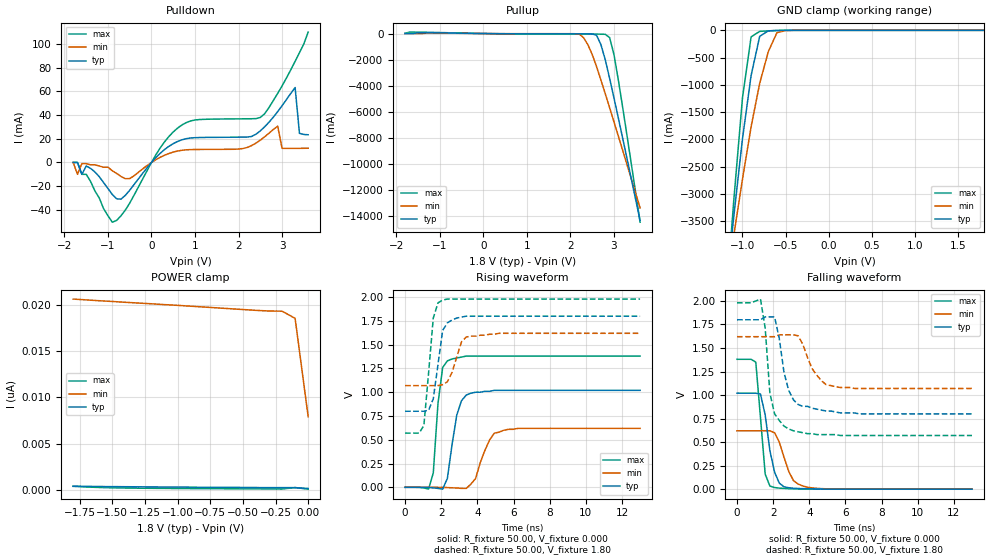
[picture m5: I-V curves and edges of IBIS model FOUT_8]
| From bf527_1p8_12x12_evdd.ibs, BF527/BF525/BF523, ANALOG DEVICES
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|   Model prw0408swcdg_3v_25
[Model]   FOUT_8
Model_type   I/O
Polarity   Non-Inverting
Enable   Active-Low
Vinl =   0.70V
Vinh =   1.00V
Vmeas =   1.20V
Cref =  50.00pF
Rref =   1.00M
Vref =  0.000V
C_comp   4.55pF   4.10pF   5.01pF
[Temperature Range]   25.00   0.12k   -40.00
[Voltage Range]   1.80V   1.62V   1.98V
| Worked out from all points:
|   slope of the pulldown table from 0 to 0.27 V, typ, clamps not added: 27.1 ohm
|   slope of the pullup table from 0 to 0.27 V, typ, clamps not added: 26.9 ohm
|   GND clamp passes 1 mA (typ) near -0.53 V on its own axis
|   rising waveform, R_fixture 50.00, V_fixture 0.000: 20-80 % time 537ps typ, 722ps min, 368ps max; typ from 0 V to 1.02 V
|   rising waveform, R_fixture 50.00, V_fixture 1.80: 20-80 % time 433ps typ, 566ps min, 388ps max; typ from 0.8 V to 1.8 V
|   falling waveform, R_fixture 50.00, V_fixture 0.000: 20-80 % time 524ps typ, 689ps min, 361ps max; typ from 1.02 V to 0 V
|   falling waveform, R_fixture 50.00, V_fixture 1.80: 20-80 % time 650ps typ, 854ps min, 454ps max; typ from 1.8 V to 0.8 V
[Pulldown]
| voltage   I(typ)   I(min)   I(max)
-1.8V     0A         0A         0A
-1.7V     0A         -10mA      0A
-1.6V     -10mA      -1mA       -10mA
-1.4V     -5mA       -2mA       -16mA
-800mV    -30.7mA    -9.3mA     -48.85mA
500mV     15.88mA    8.74mA     25.76mA
2.5V      26.66mA    18.81mA    37.95mA
2.9V      42.92mA    30.63mA    58.28mA
3V        47.86mA    11.94mA    64.57mA
3.3V      63.22mA    11.88mA    85.31mA
3.4V      24.55mA    11.91mA    92.64mA
3.6V      23.36mA    12mA       110mA
[Pullup]
| voltage   I(typ)   I(min)   I(max)
-1.8V     1.53mA     550uA      10.64mA
-1.6V     3.01mA     560uA      110mA
2.2V      -22.71mA   -39.8mA    -37.75mA
2.3V      -23.18mA   -310mA     -37.82mA
2.4V      -25.42mA   -850mA     -37.94mA
2.6V      -130mA     -2.54A     -42.67mA
2.7V      -850mA     -3.56A     -49.74mA
2.8V      -2.01A     -4.61A     -61.07mA
2.9V      -3.43A     -5.68A     -310mA
3V        -4.93A     -6.76A     -1.61A
3.1V      -6.46A     -7.85A     -3.55A
3.6V      -14.31A    -13.35A    -14.44A
[GND_clamp]
| voltage   I(typ)   I(min)   I(max)
-1.8V     -14.28A    -11.35A    -18.41A
-1.2V     -4.9A      -4.81A     -5.19A
-1.1V     -3.4A      -3.75A     -3.1A
-1V       -1.99A     -2.73A     -1.24A
-900mV    -830mA     -1.77A     -120mA
-800mV    -110mA     -970mA     -19.21mA
-700mV    -9.89mA    -390mA     -9.78mA
-600mV    -2.57mA    -42.87mA   -3.5mA
-500mV    -460uA     -4.38mA    -550uA
1.8V      170pA      19.28nA    82.46pA
[POWER_clamp]
| voltage   I(typ)   I(min)   I(max)
-1.8V     420pA      20.63nA    400pA
-1.5V     370pA      20.37nA    240pA
-1.3V     350pA      20.2nA     200pA
-400mV    270pA      19.41nA    130pA
-200mV    260pA      19.32nA    110pA
-100mV    260pA      18.55nA    270pA
0V        170pA      7.92nA     95.65pA
[Ramp]
| variable   typ   min   max
dV/dt_r   0.61/0.49n   0.37/0.70n   0.83/0.31n
dV/dt_f   0.60/0.62n   0.33/0.81n   0.84/0.40n
R_load = 50.00
[Rising Waveform]
R_fixture = 50.00
V_fixture = 0.000
V_fixture_min = 0.000
V_fixture_max = 0.000
L_fixture = 0.000H
C_fixture = 0.000F
| time   V(typ)   V(min)   V(max)
0s        0V         0V         0V
1.3ns     -1.27mV    63.15uV    -18.06mV
1.56ns    -6.38mV    20.98uV    150mV
1.82ns    -11.34mV   -220uV     880mV
2.08ns    -19.57mV   -1.01mV    1.26V
2.34ns    94.01mV    -2.97mV    1.33V
2.86ns    760mV      -6.93mV    1.36V
3.38ns    970mV      -11.91mV   1.38V
4.94ns    1.02V      570mV      1.38V
13ns      1.02V      620mV      1.38V
[Rising Waveform]
R_fixture = 50.00
V_fixture = 1.80
V_fixture_min = 1.62
V_fixture_max = 1.98
L_fixture = 0.000H
C_fixture = 0.000F
| time   V(typ)   V(min)   V(max)
0s        800mV      1.07V      570mV
780ps     800mV      1.07V      570mV
1.04ns    800mV      1.07V      650mV
1.56ns    930mV      1.07V      1.78V
1.82ns    1.29V      1.07V      1.94V
2.08ns    1.65V      1.08V      1.97V
2.34ns    1.73V      1.11V      1.98V
3.12ns    1.79V      1.53V      1.98V
3.38ns    1.8V       1.58V      1.98V
13ns      1.8V       1.62V      1.98V
[Falling Waveform]
R_fixture = 50.00
V_fixture = 0.000
V_fixture_min = 0.000
V_fixture_max = 0.000
L_fixture = 0.000H
C_fixture = 0.000F
| time   V(typ)   V(min)   V(max)
0s        1.02V      620mV      1.38V
1.04ns    1.02V      620mV      1.35V
1.3ns     1.01V      620mV      760mV
1.56ns    790mV      620mV      160mV
1.82ns    410mV      620mV      33.11mV
2.08ns    180mV      600mV      17.42mV
2.34ns    64.68mV    500mV      11.17mV
3.12ns    9.8mV      92.31mV    3.78mV
3.64ns    5.5mV      34.05mV    1.67mV
13ns      -23.45uV   6.69uV     5.6uV
[Falling Waveform]
R_fixture = 50.00
V_fixture = 1.80
V_fixture_min = 1.62
V_fixture_max = 1.98
L_fixture = 0.000H
C_fixture = 0.000F
| time   V(typ)   V(min)   V(max)
0s        1.8V       1.62V      1.98V
1.3ns     1.8V       1.62V      2.02V
1.56ns    1.83V      1.62V      1.71V
1.82ns    1.83V      1.62V      1.02V
2.08ns    1.83V      1.62V      800mV
2.86ns    1.05V      1.64V      640mV
3.38ns    900mV      1.63V      610mV
4.16ns    860mV      1.28V      590mV
4.94ns    830mV      1.11V      580mV
13ns      800mV      1.07V      570mV
